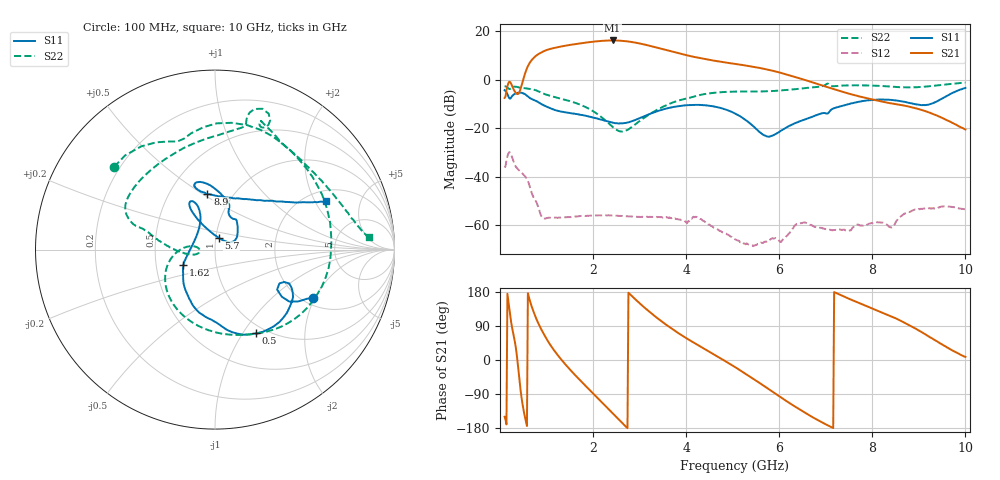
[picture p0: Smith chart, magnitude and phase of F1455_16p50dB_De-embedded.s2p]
! Integrated Device Technology
! Corporate Headquarters
! 6024 Silver Creek Valley Road
! San Jose, CA 95138  USA
! Phone:  1-408-284-8200
! Toll Free:  1-800-223-1366
! Webpage:  http://www.idt.com/
! Timing and RF Division
! 515 Groton Road, Suite 102
! Westford, MA 01886-6024
! Device:  F1455
! Description: 6-bit 0.5 dB Transmit Variable Gain Amplifier
! Frequency:  1400.0 -  2300.00 MHz
! Package:  6x6 mm Thin QFN Plastic Package: 28 pin
! State:  33
! Atten State:  16.5 dB
! Voltage:  +5.00 Volts
! Current:  217.623 mA
! Data:  The device was measured on a the F1455 evaluation board which has
!  individual transmission lines to the RF pins.  Data was collected
!  using a calibrated network analyzer.  The evaluation board was
!  de-embedded using a TRL calibration technique.
!  The reference plane is the edge of the package pin.
!  Pin  1 = CSb
!  Pin  2 = DATA
!  Pin  3 = CLK
!  Pin  4 = RSET
!  Pin  5 = GND
!  Pin  6 = RFIN  = Port 1
!  Pin  7 = GND
!  Pin  8 = NC
!  Pin  9 = NC
!  Pin 10 = NC
!  Pin 11 = NC
!  Pin 12 = NC
!  Pin 13 = NC
!  Pin 14 = /STBY
!  Pin 15 = GND
!  Pin 16 = RFOUT  = Port 2
!  Pin 17 = GND
!  Pin 18 = NC
!  Pin 19 = NC
!  Pin 20 = NC
!  Pin 21 = GND
!  Pin 22 = NC
!  Pin 23 = GND
!  Pin 24 = NC
!  Pin 25 = NC
!  Pin 26 = NC
!  Pin 27 = GND
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# GHz S dB R 50
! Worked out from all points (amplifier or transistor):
!   496 points, 100 MHz to 10 GHz, reference 50 ohm
!   highest |S21| = 16.1 dB at 2.42 GHz (marker M1)
!   |S21| within 3 dB of that: 1.186 GHz to 3.386 GHz (2.2 GHz wide, 96.2 % of centre)
!   unconditionally stable (mu >= 1): start of sweep to end of sweep
!   at 1.74 GHz: K = 50.90, MAG = 15.6 dB, |S12| = -56.3 dB
!   at 5.06 GHz: K = 307.97, MAG = 8.3 dB, |S12| = -65.9 dB
!   at 10 GHz: K = 353.59, MAG = -12.0 dB, |S12| = -53.6 dB
!   S11 on the Smith chart (normalised r, x): 100 MHz: 2.25, -1.92; 500 MHz: 0.90, -1.15; 1.62 GHz: 0.69, -0.13; 5.7 GHz: 1.03, +0.14; 8.9 GHz: 0.76, +0.53; 10 GHz: 2.48, +2.47
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0.1  -4.35 -26.3  -7.55 -149.7  -36.29 46.4  -2.77 140.7
0.26  -6.86 -24.5  -2.59 85.8  -32.03 -76.4  -3.29 95.6
0.38  -5.46 -41.4  -5.99 -5.9  -36.84 -115.5  -3.10 57.6
0.5  -5.68 -63.8  0.12 -127.6  -39.05 -153.8  -3.47 27.4
0.68  -7.98 -91.0  7.99 142.0  -46.58 142.0  -3.93 -14.0
0.82  -9.27 -109.1  10.44 97.8  -52.43 117.5  -4.78 -45.4
0.96  -10.80 -123.2  11.87 64.6  -57.33 125.2  -5.96 -70.6
1.28  -13.08 -142.9  13.53 6.9  -56.91 97.3  -7.73 -114.2
1.62  -14.13 -153.7  14.65 -40.5  -56.46 68.5  -9.60 -146.8
1.76  -14.58 -157.6  15.04 -58.3  -56.21 58.0  -10.63 -157.8
2.1  -16.11 -169.0  15.83 -100.4  -55.99 38.1  -14.31 179.9
2.42  -17.73 170.6  16.14 -140.4  -56.05 21.9  -19.49 171.7
2.8  -17.38 135.4  15.59 172.8  -56.44 7.0  -19.99 -166.8
3.1  -15.11 117.8  14.47 138.8  -56.70 -1.7  -15.79 -172.3
3.4  -12.92 112.1  13.07 108.7  -56.64 -12.1  -12.23 177.7
4.08  -10.48 115.5  9.73 51.9  -57.85 -25.5  -7.46 163.7
5.06  -14.05 119.8  6.45 -19.4  -65.94 -67.0  -4.95 148.7
5.7  -23.13 73.5  4.34 -70.8  -66.83 -37.4  -4.84 122.5
6.7  -15.41 41.9  -1.04 -149.7  -60.08 -131.6  -3.24 78.7
8.36  -8.31 107.0  -9.66 117.3  -60.68 131.6  -2.83 62.7
8.9  -10.08 97.7  -11.65 84.7  -53.70 129.8  -3.18 41.2
10  -3.42 23.7  -20.58 8.3  -53.56 49.6  -1.28 4.7
